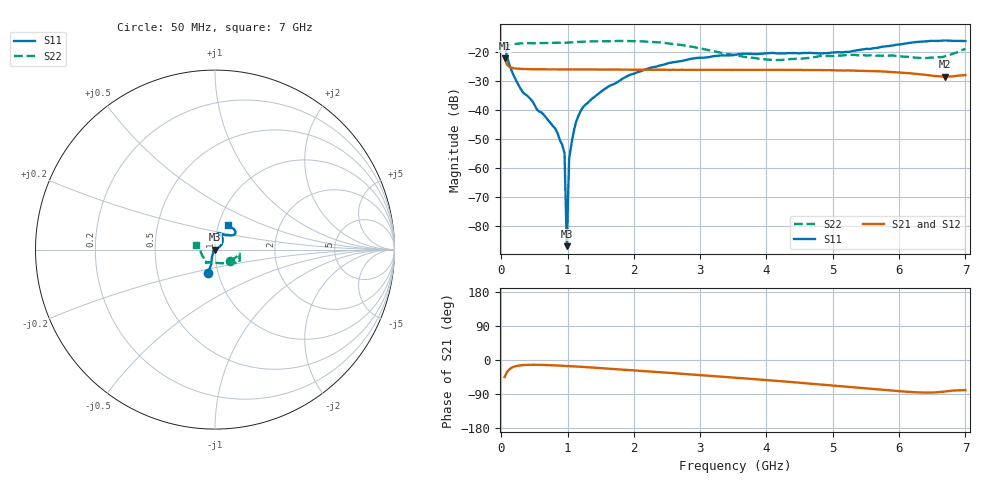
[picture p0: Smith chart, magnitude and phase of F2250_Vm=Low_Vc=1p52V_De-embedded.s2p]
! Integrated Device Technology
! Corporate Headquarters
! 6024 Silver Creek Valley Road
! San Jose, CA 95138  USA
! Phone:  1-408-284-8200
! Toll Free:  1-800-223-1366
! Webpage:  http://www.idt.com/
! Timing and RF Division
! 515 Groton Road, Suite 102
! Westford, MA 01886-6024
! Device:  F2250
! Description: Voltage Variable RF Attenuator
! Frequency:  50.0 -  6000.00 MHz
! Package:  3x3 mm Thin QFN Plastic Package: 16 pin
! Ports:  2 RF, 3 DC
!  Pin  1  = GND
!  Pin  2  = NC
!  Pin  3  = RF1  = Port 1
!  Pin  4  = NC
!  Pin  5  = GND
!  Pin  6  = GND
!  Pin  7  = GND
!  Pin  8  = GND
!  Pin  9  = NC
!  Pin 10  = RF2  = Port 2
!  Pin 11  = NC
!  Pin 12  = GND
!  Pin 13  = GND
!  Pin 14  = VCNTRL
!  Pin 15  = VDD
!  Pin 16  = VMODE
! Vcntrl:  1.520 Volts
! Vmode:  +0.000 Volts
! Vdd:  +3.30  Volts
! Current:  1.190 mA
! Data:  The device was measured on a the F2250 evaluation board which has
!  individual transmission lines to the RF pins.  Data was collected
!  using a calibrated network analyzer.  The evaluation board was
!  de-embedded using a TRL calibration technique.
!  The reference plane is the edge of the package pin.
! Misc:  SN 10
!  Action Tracker AT0258
! Date Measured:  2014-11-26
! Date:  2015-10-15  MJV
! Note:
!  Integrated Device Technology supplies this data as a sample of measured
!  data at the package pin for this product.  Your particular data for this
!  product may vary.
!  Data was taken at 25 degrees C.
!  Integrated Device Technology reserves the right to change this data at anytime.
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# GHz S dB R 50
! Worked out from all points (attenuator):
!   201 points, 50 MHz to 7 GHz, reference 50 ohm
!   highest |S21| = -22.28 dB at 50 MHz (marker M1); lowest = -28.6 dB at 6.687 GHz (marker M2)
!   lowest |S11| = -87.0 dB at 988.2 MHz (marker M3), VSWR 1.00, Z = 50 + j0.00434 ohm
!   |S11| at or under -10 dB: start of sweep to end of sweep
!   |S22| runs from -22.9 to -16.3 dB; largest |S21 - S12| = 0.00026
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0.05  -17.21 -106.5  -22.28 -45.0  -22.29 -45.0  -19.31 -37.1
0.1195  -24.35 -107.8  -25.19 -24.9  -25.20 -24.9  -17.66 -12.4
0.29325  -32.88 -118.4  -25.91 -14.0  -25.93 -14.0  -17.13 -9.6
0.8145  -46.51 -179.5  -26.12 -14.3  -26.12 -14.3  -16.96 -16.0
0.91875  -52.06 151.4  -26.14 -15.2  -26.14 -15.2  -16.90 -18.0
0.9535  -54.97 -172.2  -26.13 -15.4  -26.16 -15.4  -16.95 -18.3
0.98825  -87.02 76.5  -26.14 -15.8  -26.16 -15.7  -16.88 -18.7
1.023  -56.86 17.0  -26.15 -16.1  -26.15 -16.1  -16.83 -18.8
1.0925  -47.55 21.5  -26.13 -16.7  -26.13 -16.7  -16.77 -19.9
1.12725  -44.26 23.3  -26.12 -17.1  -26.13 -17.1  -16.70 -20.5
1.2315  -39.15 24.1  -26.13 -18.2  -26.14 -18.2  -16.53 -22.2
1.5095  -33.67 29.5  -26.14 -21.5  -26.15 -21.5  -16.43 -24.6
1.857  -28.95 34.3  -26.21 -25.7  -26.16 -25.7  -16.31 -27.8
2.37825  -24.86 43.3  -26.22 -32.1  -26.23 -32.0  -16.79 -31.6
2.93425  -22.20 57.3  -26.29 -39.0  -26.26 -39.0  -18.57 -38.9
3.525  -21.08 70.7  -26.27 -46.7  -26.26 -46.7  -21.23 -61.2
4.11575  -20.46 78.5  -26.28 -54.6  -26.26 -54.6  -22.90 -93.1
4.7065  -20.49 71.4  -26.34 -63.0  -26.34 -63.0  -21.90 -116.4
5.85325  -18.00 39.4  -26.95 -80.2  -26.94 -80.2  -21.35 -128.9
6.3745  -16.47 40.7  -27.94 -85.9  -27.96 -86.0  -22.25 -147.7
6.68725  -16.13 48.2  -28.65 -83.2  -28.66 -83.2  -21.59 -176.3
7  -16.32 62.8  -28.03 -79.3  -27.99 -79.4  -19.01 165.5
